(* Logix 5000 AddOnInstructionDefinition export VLT_EIP_FC_BASIC; software revision 31.00 *)

ADD_ON_INSTRUCTION VLT_EIP_FC_BASIC   (* revision 1.0, vendor Danfoss Drives *)
// Basic control Add-On instruction for Danfoss FC series Drives
VAR_INPUT
   DRV_EN : BOOL; {visible}   // Enable Drive
   RUN : BOOL; {visible}   // Start the motor
   REVERSE : BOOL; {visible}   // Reverse motor direction
   REF_VALUE : INT; {visible}   // Drive ref. 0-10000 = 0 - 100.00%
   RESET : BOOL; {visible}   // Resets alarm
   COMM_STATUS : BOOL; {required}   // Communication status
END_VAR
VAR_OUTPUT
   READY : BOOL; {access Read Only, visible}   // Ready for operation
   FAULT : BOOL; {access Read Only, visible}   // Alarm pending
   WARNING : BOOL; {access Read Only, visible}   // Warning pending
   RUNNING : BOOL; {access Read Only, visible}   // Motor engaged
   RUN_ON_REF : BOOL; {access Read Only, visible}   // Speed = reference
   COMM_OK : BOOL; {access Read Only, visible}   // Communication OK
   MAV : INT; {access Read Only, visible}   // Main actual value
   MOTORCURRENT : REAL; {access Read Only, visible}   // Motor current in Amps
END_VAR
VAR_IN_OUT
   PCDREAD : INT[4]; {required}   // Process data from Drive
        [0]   // Status word
        [1]   // Main actual value
        [2]   // Motor current (LSW)
        [3]   // Motor current (MSW)
   PCDWRITE : INT[2]; {required}   // Process data to Drive
        [0]   // Control word
        [1]   // Main reference value
END_VAR
VAR
   MRV : INT; {access None}   // Internal variable. Holds Main reference value
   MOTORCURRENT_DINT : DINT; {access None}   // Internal variable - Motor current raw value (without scaling)
END_VAR

ROUTINE Logic   (* structured text *)
   (*
   DANFOSS DRIVES - Fieldbus and System Integration (R & D)
   
   Specification:
   VLT Drives - Basic drive operation - "DD_VLT_EIP_BASIC" function block through Cyclic communication
   This function block has been designed to work with FC profile.
   
   *)
   (* Start of the program *)
   (* Mapping Outputs *)
   COMM_OK := NOT COMM_STATUS;															(* 1 = The communication between Device and PLC is healthy *)
   READY := (PCDREAD[0].0 & 															(* 1 = Control Ready *)
   		  PCDREAD[0].1 & 															(* 1 = Frequency converter ready *)
   		  PCDREAD[0].2 & 															(* 1 = Costing stop *)
   		  PCDREAD[0].9) &															(* 1 = Bus control *)
   		  COMM_OK;																	(* 1 = Communication between device and PLC is healthy *)
   FAULT := (PCDREAD[0].3 OR 															(* 1 = The frequency converter trips *)
   		  PCDREAD[0].4 OR	  														(* 1 = The frequency converter shows an error but does not trip. *)
   		  PCDREAD[0].6 OR	  														(* 1 = The frequency converter is tripped and locked *)
   		  NOT COMM_OK);																(* 1 = Communication failure *)
   WARNING := PCDREAD[0].7 & COMM_OK;  												(* 1 = A warning has occurred on the drive *)
   RUNNING := PCDREAD[0].11 & COMM_OK; 												(* 1 = The frequency converter has a start signal or the output frequency is and greater than 0 Hz.*)
   RUN_ON_REF := PCDREAD[0].8 AND COMM_OK;												(* 1 = The actual motor speed reaches the preset speed reference *)
   IF COMM_OK THEN
   	COP(PCDREAD[2],MOTORCURRENT_DINT,2);											(* Converting SINT to DINT - MotorCurrent *)
   	MOTORCURRENT := MOTORCURRENT_DINT/100.0;										(* Motor scaling in Amps *)
   	MAV := (PCDREAD[1] * 10000)/16384;												(* Motor actual Speed in integer format *)
   END_IF;
   (* Control Word Mapping *)
   PCDWRITE[0].0 := 0;																	(* Selection of Preset reference value– PRESET_REF_1 and PRESET_REF_2 are used to choose between the four reference values which are pre-programmed in Parameter 3-10 Preset Reference *)
   PCDWRITE[0].1 := 0;																	(* Selection of Preset reference value– PRESET_REF_1 and PRESET_REF_2 are used to choose between the four reference values which are pre-programmed in Parameter 3-10 Preset Reference *)
   PCDWRITE[0].2 := DRV_EN;															(* 0 = DC brake; 1 = Ramp *)
   PCDWRITE[0].3 := DRV_EN;															(* 0 = No coasting; 1 = Enables the frequency converter to start the motor if the other starting conditions have been fulfilled *)
   PCDWRITE[0].4 := DRV_EN;															(* 0 = Quickstop; 1 = Enables the frequency converter ramp the motor speed down to stop *)
   PCDWRITE[0].5 := DRV_EN;															(* 0 = Hold output frequency; 1 = Uses Ramp *)
   PCDWRITE[0].6 := RUN AND (NOT FAULT);												(* 0 = Stop; 1 = Start *)
   PCDWRITE[0].7 := RESET;					 											(* 0 = No function; 1 = Reset command *)
   PCDWRITE[0].8 := 0;																	(* 0 = No function, 1 = Jog *)
   PCDWRITE[0].9 := 0;																	(* 0 = Ramp 1, 1 = Ramp 2 *)
   PCDWRITE[0].10:= 1;																	(* 0 = Ignore CTW; 1 = Data Valid *)
   PCDWRITE[0].11 := 0;																(* 0 = Relay 01 deactived, 1 = Relay 01 active *)
   PCDWRITE[0].12 := 0;																(* 0 = Relay 04 deactived, 1 = Relay 04 active *)
   PCDWRITE[0].13 := 0;																(* 0 = Parameter set-up, 1 = selection lsb *)
   PCDWRITE[0].14 := 0;																(* 0 = Parameter set-up, 1 = selection msb *)
   PCDWRITE[0].15 := REVERSE;															(* 0 = No Reverse, 1 = Reverse *)
   (* Set the Motor reference - Capping Reference between 0 to 100 *)
   IF REF_VALUE > 10000 then
   	MRV := 10000;																	(* High Limit *)
   ELSIF REF_VALUE <=0 then
   	MRV  := 0;																		(* Low Limit *)
   ELSE
   	MRV := REF_VALUE;
   END_IF;
   PCDWRITE[1] := ((MRV * 16384) /10000);												(* Writing MRV value to frequency converter *)
   (* End of the program *)
END_ROUTINE
END_ADD_ON_INSTRUCTION
